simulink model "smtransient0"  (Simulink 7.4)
settings: Solver=ode45  StartTime=0.0  StopTime=5  MaxStep=1e-3  RelTol=1e-4  AbsTol=1e-4
PreLoadFcn:
  | clc
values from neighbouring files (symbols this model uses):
  Bm = 0.10    (= 0.1)    [IMabc2.m]    (also in imabcparam.m = 0.01; IMabcrun0.m = 0.01; IMabcrun1.m = 0.001; IMcur0.m = 1e-06)
  H = 0.60    (= 0.6)    [IMabc2.m]    (also in IMcur0.m = 0.3; imdef0vec.m = 0.3; imdef1vec.m = 0.3; imdef2vec.m = 0.3)
  n0 = 0.98    [imdef0vec.m]    (also in imdef1vec.m = 0.978; imdef2vec.m; imdefrotflux.m; imdefSIvec1.m = 0.95)
  Ra = .95    (= 0.95)    [altwdgs.m]    (also in Ccurverun.m = 0.018)
  tc = abs(fco)    [im3phase.m]
  Te0 = 0.75/wo*p*(Is*conj(Is)*Req)    [imdefSIvec1.m]
  V = [Vas 0 0].'    [Actac.m]    (also in acttrcalc1.m = str2num(get(h,'string')); im3d.m = eval(get(hVs,'String')); IMabc2.m = [vas vbs vcs 0 0 0]'; IMabcf0.m = [vas vbs vcs 0 0 0]')
  wo = 2*pi*freq0    [calc0.m]    (also in IMabc2.m = 376.991118431; imabcparam.m = 376.991118431; IMabcrun0.m = 376.991118431; IMabcrun1.m = 376.991118431)
undefined symbols (not defined in the file or in its folder): delta0, fa0, fk0, Lal, Lfl, Lkdl, Lkql, Lmd, Lmq, phif0, Rf, Rkd, Rkq, vf0

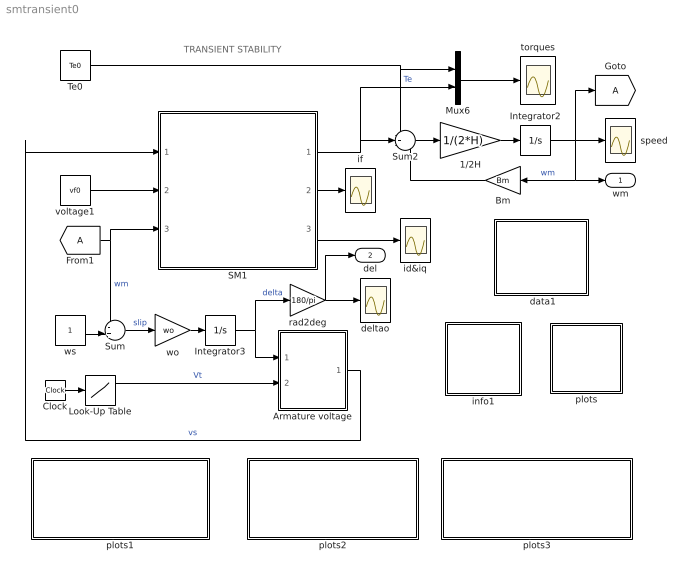
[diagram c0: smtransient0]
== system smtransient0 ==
  note: TRANSIENT STABILITY
  " data1" : Subsystem
  1/2H : Gain  Gain=1/(2*H)  ParameterDataType=sfix(16)  ParameterScaling=2^0  OutDataType=sfix(16)  OutScaling=2^0
  Armature voltage : Subsystem
  Bm : Gain  Gain=Bm  ParameterDataType=sfix(16)  ParameterScaling=2^0  OutDataType=sfix(16)  OutScaling=2^0
  Clock : Clock
  Integrator2 : Integrator  InitialCondition=n0
  Integrator3 : Integrator  InitialCondition=delta0
  Look-Up Table : Lookup  InputValues=[0 0.5 0.5 0.5+tc 0.5+tc 3]  Table=[V V 0 0 V V]  OutDataType=sfix(16)  OutScaling=2^0
  Mux6 : Mux  Inputs=2
  SM1 : Subsystem
  Sum : Sum  Inputs=-+|  OutDataType=sfix(16)  OutScaling=2^0
  Sum2 : Sum  Inputs=-+-  OutDataType=sfix(16)  OutScaling=2^0
  Te0 : Constant  Value=Te0  OutDataType=sfix(16)  OutScaling=2^0
  deltao : Scope
  id&iq : Scope
  if : Scope
  info1 : Subsystem
  plots : Subsystem
  plots1 : Subsystem
  plots2 : Subsystem
  plots3 : Subsystem
  rad2deg : Gain  Gain=180/pi  ParameterDataType=sfix(16)  ParameterScaling=2^0  OutDataType=sfix(16)  OutScaling=2^0
  speed : Scope
  torques : Scope
  voltage1 : Constant  Value=vf0  OutDataType=sfix(16)  OutScaling=2^0
  wo : Gain  Gain=wo  ParameterDataType=sfix(16)  ParameterScaling=2^0  OutDataType=sfix(16)  OutScaling=2^0
  ws : Constant  OutDataType=sfix(16)  OutScaling=2^0
  wm : Outport
  del : Outport  Port=2
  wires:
  Mux6/1 -> torques/1
  voltage1/1 -> SM1/2(vf)
  SM1/2(if) -> if/1
  Sum2/1 -> 1/2H/1
  1/2H/1 -> Integrator2/1
  SM1/1(Te) -> Sum2/2, Mux6/2  "Te"
  Bm/1 -> Sum2/3
  Integrator2/1 -> speed/1, [A], Bm/1, wm/1  "wm"
  Te0/1 -> Mux6/1, Sum2/1
  ws/1 -> Sum/2
  Sum/1 -> wo/1  "slip"
  wo/1 -> Integrator3/1
  Armature voltage/1(vs) -> SM1/1(vs)  "vs"
  Integrator3/1 -> Armature voltage/1(delta), rad2deg/1  "delta"
  SM1/3(ia) -> id&iq/1
  rad2deg/1 -> deltao/1, del/1
  Clock/1 -> Look-Up Table/1
  Look-Up Table/1 -> Armature voltage/2(Vt)  "Vt"
  [A] -> SM1/3(wm), Sum/1  "wm"

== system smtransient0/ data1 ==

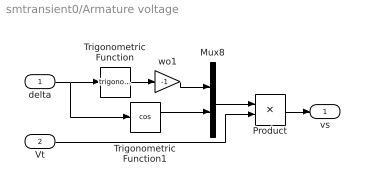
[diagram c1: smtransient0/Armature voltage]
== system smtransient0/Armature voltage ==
  delta : Inport  OutDataType=sfix(16)  OutScaling=2^0
  Vt : Inport  Port=2  OutDataType=sfix(16)  OutScaling=2^0
  Mux8 : Mux  Inputs=2
  Product : Product  OutDataType=sfix(16)  OutScaling=2^0
  Trigonometric Function : Trigonometry
  Trigonometric Function1 : Trigonometry  Operator=cos
  wo1 : Gain  Gain=-1  ParameterDataType=sfix(16)  ParameterScaling=2^0  OutDataType=sfix(16)  OutScaling=2^0
  vs : Outport
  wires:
  delta/1 -> Trigonometric Function/1, Trigonometric Function1/1
  Trigonometric Function/1 -> wo1/1
  Mux8/1 -> Product/1
  wo1/1 -> Mux8/1
  Trigonometric Function1/1 -> Mux8/2
  Product/1 -> vs/1
  Vt/1 -> Product/2

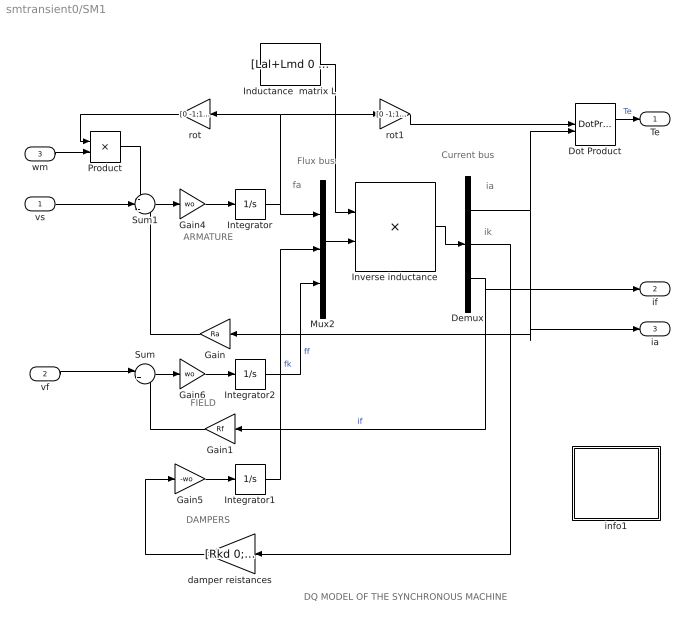
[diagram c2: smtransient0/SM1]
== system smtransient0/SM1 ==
  note: DAMPERS
  note: ARMATURE
  note: fa
  note: ia
  note: FIELD
  note: DQ MODEL OF THE SYNCHRONOUS MACHINE
  note: Flux bus
  note: Current bus
  note: ik
  vs : Inport  OutDataType=sfix(16)  OutScaling=2^0
  vf : Inport  Port=2  OutDataType=sfix(16)  OutScaling=2^0
  wm : Inport  Port=3  OutDataType=sfix(16)  OutScaling=2^0
  Demux : Demux  Outputs=3
  Dot Product : DotProduct  OutDataType=fixdt(1, 16)  OutScaling=2^-10
  Gain : Gain  Gain=Ra  ParameterDataType=sfix(16)  ParameterScaling=2^0  OutDataType=sfix(16)  OutScaling=2^0
  Gain1 : Gain  Gain=Rf  ParameterDataType=sfix(16)  ParameterScaling=2^0  OutDataType=sfix(16)  OutScaling=2^0
  Gain4 : Gain  Gain=wo  ParameterDataType=sfix(16)  ParameterScaling=2^0  OutDataType=sfix(16)  OutScaling=2^0
  Gain5 : Gain  Gain=-wo  ParameterDataType=sfix(16)  ParameterScaling=2^0  OutDataType=sfix(16)  OutScaling=2^0
  Gain6 : Gain  Gain=wo  ParameterDataType=sfix(16)  ParameterScaling=2^0  OutDataType=sfix(16)  OutScaling=2^0
  Inductance  matrix L : Constant  Value=[Lal+Lmd 0 Lmd 0 Lmd;0 Lal+Lmq 0 Lmq 0;Lmd 0 Lmd+Lkdl 0 Lmd;0 Lmq 0 Lmq+Lkql 0;Lmd 0 Lmd 0 Lmd+Lfl]  VectorParams1D=off  OutDataType=fixdt(1, 16)  OutScaling=2^0
  Integrator : Integrator  InitialCondition=fa0
  Integrator1 : Integrator  InitialCondition=fk0
  Integrator2 : Integrator  InitialCondition=phif0
  Inverse inductance : Product  Inputs=/*  Multiplication=Matrix(*)  OutDataType=sfix(16)  OutScaling=2^0
  Mux2 : Mux  Inputs=3
  Product : Product  OutDataType=sfix(16)  OutScaling=2^0
  Sum : Sum  Inputs=|+-  OutDataType=sfix(16)  OutScaling=2^0
  Sum1 : Sum  Inputs=-+-  OutDataType=sfix(16)  OutScaling=2^0
  damper reistances : Gain  Gain=[Rkd 0;0 Rkq]  Multiplication=Matrix(K*u)  ParameterDataType=sfix(16)  ParameterScaling=2^0  OutDataType=sfix(16)  OutScaling=2^0
  info1 : Subsystem
  rot : Gain  Gain=[0 -1;1 0]  Multiplication=Matrix(K*u)  ParameterDataType=sfix(16)  ParameterScaling=2^0  OutDataType=sfix(16)  OutScaling=2^0
  rot1 : Gain  Gain=[0 -1;1 0]  Multiplication=Matrix(K*u)  ParameterDataType=sfix(16)  ParameterScaling=2^0  OutDataType=sfix(16)  OutScaling=2^0
  Te : Outport
  if : Outport  Port=2
  ia : Outport  Port=3
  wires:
  Product/1 -> Sum1/1
  rot/1 -> Product/1
  wm/1 -> Product/2
  Gain5/1 -> Integrator1/1
  damper reistances/1 -> Gain5/1
  Integrator/1 -> Mux2/1, rot/1, rot1/1
  Sum1/1 -> Gain4/1
  Gain4/1 -> Integrator/1
  vs/1 -> Sum1/2
  Gain/1 -> Sum1/3
  Gain6/1 -> Integrator2/1
  Sum/1 -> Gain6/1
  vf/1 -> Sum/1
  Gain1/1 -> Sum/2
  rot1/1 -> Dot Product/1
  Demux/1 -> Gain/1, ia/1, Dot Product/2
  Dot Product/1 -> Te/1  "Te"
  Integrator1/1 -> Mux2/2  "fk"
  Integrator2/1 -> Mux2/3  "ff"
  Demux/2 -> damper reistances/1
  Demux/3 -> if/1, Gain1/1  "if"
  Mux2/1 -> Inverse inductance/2
  Inductance  matrix L/1 -> Inverse inductance/1
  Inverse inductance/1 -> Demux/1

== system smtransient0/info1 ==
  note: Synchronous machine transient stability
  note: This demonstration illustrates the dynamics of a synchronous machine following the sudden application and removal of a three-phase short circuit at the terminals. Four models of the synchronous machine are provided: 1) A complete model (5th-order) 2) Armature transients ignored by setting dfa/dt=0 (3rd-order) 3) Both armature transients and damper effects are neglected (1st-order) 4) Constant field flux linkage (zero-order) Click the DATA block to enter the parameters and prefault operating conditions. Initialize and then Start the simulation.

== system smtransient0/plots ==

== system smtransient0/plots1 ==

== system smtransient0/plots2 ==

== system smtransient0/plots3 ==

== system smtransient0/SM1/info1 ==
  note: This demonstration illustrates the dynamics of a synchronous generator, initially at no load, following a three-phase short circuit at the terminals.
  note: Synchronous machine transients under shortcircuit
